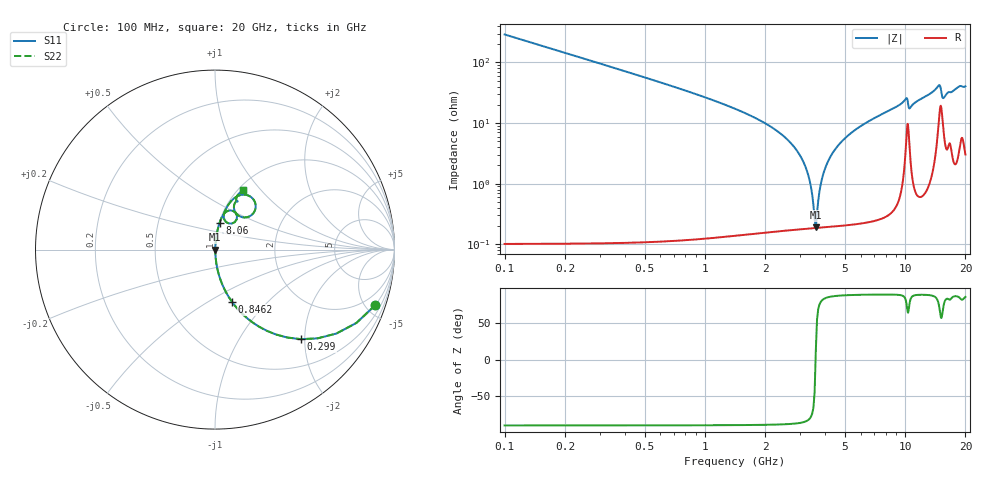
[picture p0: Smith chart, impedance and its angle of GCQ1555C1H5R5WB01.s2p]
!Murata Part Number: GCQ1555C1H5R5WB01
!These Parameters are Measured in Series Mode Connection
!Data Generated on Jan 08, 2026
!  o--ll--o
!Port1  Port2
!  o------o
!Operation Temp=25[degC], DC Bias Voltage=0[V]
!Freq. Start=100[MHz] Stop=20[GHz] 401[Steps]
# Hz S RI R 50
!Freq.(Hz) S11(Real) S11(Imag) S21(Real) S21(Imag) S12(Real) S12(Imag) S22(Real) S22(Imag)
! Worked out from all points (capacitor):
!   401 points, 100 MHz to 20 GHz, reference 50 ohm
!   read as one part in series: C = 5.5 pF near 199.5 MHz
!   lowest |Z| = 191 mohm at 3.583 GHz (marker M1)
!   series resonance near 3.573 GHz, so ESL is about 360 pH
!   S11 on the Smith chart (normalised r, x): 100 MHz: 1.00, -5.78; 299 MHz: 1.00, -1.92; 846.2 MHz: 1.00, -0.65; 8.06 GHz: 1.01, +0.31; 20 GHz: 1.06, +0.81
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1e8  0.8931 -0.3088  0.1069 0.3088  0.1069 0.3088  0.8931 -0.3088
2.99e8  0.4801 -0.4991  0.5199 0.4991  0.5199 0.4991  0.4801 -0.4991
5.4775e8  0.2106 -0.4067  0.7894 0.4067  0.7894 0.4067  0.2106 -0.4067
8.4625e8  0.0951 -0.2916  0.9049 0.2916  0.9049 0.2916  0.0951 -0.2916
1.5925e9  0.0221 -0.142  0.9779 0.142  0.9779 0.142  0.0221 -0.142
2.83625e9  0.00315 -0.0376  0.9968 0.0376  0.9968 0.0376  0.00315 -0.0376
3.23425e9  0.00206 -0.0161  0.9979 0.0161  0.9979 0.0161  0.00206 -0.0161
3.43325e9  0.00188 -0.00645  0.9981 0.00645  0.9981 0.00645  0.00188 -0.00645
3.53275e9  0.00185 -0.00183  0.9981 0.00183  0.9981 0.00183  0.00185 -0.00183
3.5825e9  0.00186 0.000428  0.9981 -0.000428  0.9981 -0.000428  0.00186 0.000428
3.93075e9  0.00214 0.0155  0.9979 -0.0155  0.9979 -0.0155  0.00214 0.0155
4.42825e9  0.0032 0.035  0.9968 -0.035  0.9968 -0.035  0.0032 0.035
5.32375e9  0.00652 0.0663  0.9935 -0.0663  0.9935 -0.0663  0.00652 0.0663
6.7665e9  0.0149 0.111  0.9851 -0.111  0.9851 -0.111  0.0149 0.111
8.06e9  0.0255 0.1484  0.9745 -0.1484  0.9745 -0.1484  0.0255 0.1484
1.005e10  0.0845 0.218  0.9155 -0.218  0.9155 -0.218  0.0845 0.218
1.05475e10  0.0602 0.1558  0.9398 -0.1558  0.9398 -0.1558  0.0602 0.1558
1.338325e10  0.095 0.2755  0.905 -0.2755  0.905 -0.2755  0.095 0.2755
1.49255e10  0.2264 0.2495  0.7736 -0.2495  0.7736 -0.2495  0.2264 0.2495
1.5423e10  0.1323 0.1886  0.8677 -0.1886  0.8677 -0.1886  0.1323 0.1886
1.67165e10  0.1264 0.268  0.8736 -0.268  0.8736 -0.268  0.1264 0.268
2e10  0.1585 0.3296  0.8415 -0.3296  0.8415 -0.3296  0.1585 0.3296
